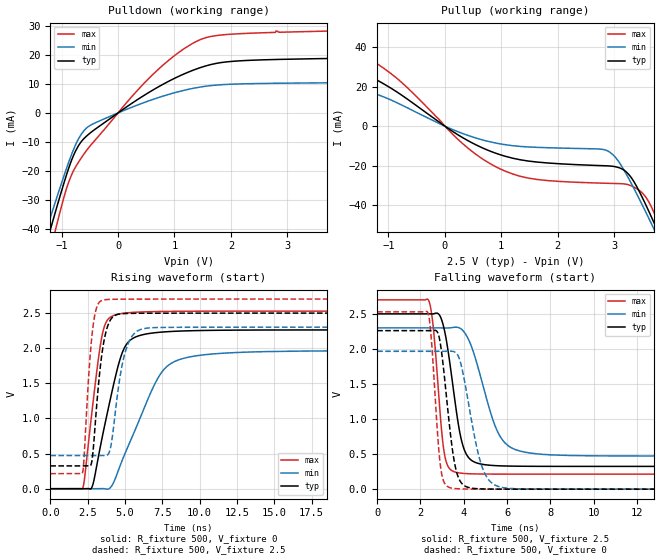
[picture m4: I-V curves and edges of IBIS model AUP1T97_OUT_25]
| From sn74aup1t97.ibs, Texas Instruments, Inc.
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[Model]   AUP1T97_OUT_25
Model_type  Output
Vref =   0
Rref =   1E6
Cref =   30p
Vmeas =   1.25
| variable   typ   min   max
C_comp   2.77pF   1.87pF   4.14pF
| C_pullup   3.12pF   1.87pF   4.14pF
| C_pulldown   2.42pF   2.13pF   2.99pF
[Temperature Range]   40   100   -40
| Ambient temperature   25   85   -40
[Voltage range]   2.5   2.3   2.7
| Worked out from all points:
|   slope of the pulldown table from 0 to 0.375 V, typ, clamps not added: 75.2 ohm
|   slope of the pullup table from 0 to 0.375 V, typ, clamps not added: 55.1 ohm
|   rising waveform, R_fixture 500, V_fixture 0: 20-80 % time 1.4ns typ, 2.41ns min, 859ps max; typ from 0 V to 2.26 V
|   falling waveform, R_fixture 500, V_fixture 2.5: 20-80 % time 621ps typ, 1.07ns min, 392ps max; typ from 2.5 V to 0.325 V
|   rising waveform, R_fixture 500, V_fixture 2.5: 20-80 % time 611ps typ, 791ps min, 469ps max; typ from 0.325 V to 2.5 V
|   falling waveform, R_fixture 500, V_fixture 0: 20-80 % time 497ps typ, 750ps min, 332ps max; typ from 2.26 V to 0 V
[Pulldown]
| AUP1T97_OUT_25
|   Voltage   I(typ)   I(min)   I(max)
-3.6V     -214mA     -193.5mA   -239.7mA
-1.26V    -44.55mA   -39.92mA   -52.42mA
-1.205V   -40.74mA   -36.52mA   -48.02mA
-1.115V   -34.57mA   -31.02mA   -40.91mA
-800mV    -15.22mA   -13.22mA   -20.4mA
-685mV    -10.84mA   -8.445mA   -16.54mA
-540mV    -7.689mA   -4.911mA   -12.5mA
675mV     8.558mA    5.038mA    14.35mA
1.105V    12.9mA     7.5mA      21.28mA
1.52V     16.03mA    9.129mA    25.76mA
2.585V    18.34mA    10.19mA    27.69mA
7.2V      19.61mA    10.73mA    29.61mA
[Pullup]
| AUP1T97_OUT_25
|   Voltage   I(typ)   I(min)   I(max)
-3.6V     37.28mA    23.5mA     50.35mA
-2.355V   24.65mA    15.21mA    35.57mA
-1.425V   26.01mA    17.2mA     35.58mA
-760mV    15.58mA    10.63mA    21.96mA
405mV     -7.279mA   -4.651mA   -11.04mA
1.05V     -15.07mA   -9.293mA   -22.54mA
2.845V    -20.04mA   -12.07mA   -28.88mA
3.17V     -22.17mA   -22.09mA   -29.2mA
3.455V    -33.67mA   -37.48mA   -32.73mA
3.685V    -47.61mA   -50.92mA   -42.5mA
3.82V     -56.28mA   -59.04mA   -51.47mA
7.2V      -294.7mA   -278.7mA   -311.5mA
[Ramp]
| AUP1T97_OUT_25
| variable   typ   min   max
dV/dt_r   1.36/1.41E-09   1.18/2.41E-09   1.52/8.61E-10
dV/dt_f   1.31/6.28E-10   1.10/1.07E-09   1.50/3.97E-10
R_load = 500
[Rising Waveform]
| AUP1T97_OUT_25
R_fixture =   500
C_fixture =   0
L_fixture =   0
V_fixture =   0
V_fixture_min = 0
V_fixture_max = 0
|   Time   V(typ)   V(min)   V(max)
0s        19.04nV    76.96nV    1.464nV
2.18ns    -12.02uV   435.7nV    11.67mV
2.81ns    31.98mV    -14uV      1.128V
3.435ns   685.6mV    1.468mV    2.14V
4.315ns   1.55V      122.9mV    2.471V
4.86ns    1.956V     425.6mV    2.497V
5.43ns    2.126V     710.7mV    2.509V
7.33ns    2.227V     1.616V     2.523V
8.865ns   2.245V     1.853V     2.526V
34.99ns   2.261V     1.966V     2.528V
[Falling Waveform]
| AUP1T97_OUT_25
R_fixture =   500
C_fixture =   0
L_fixture =   0
V_fixture =   2.5
V_fixture_min = 2.3
V_fixture_max = 2.7
|   Time   V(typ)   V(min)   V(max)
0s        2.5V       2.3V       2.7V
2.38ns    2.5V       2.3V       2.69V
2.595ns   2.5V       2.3V       2.298V
3.09ns    2.288V     2.299V     534.1mV
3.665ns   1.094V     2.309V     238.6mV
3.96ns    620.3mV    2.262V     225.5mV
4.33ns    416.9mV    2.055V     219mV
5.585ns   333.8mV    804.4mV    214.8mV
6.815ns   326.6mV    528.2mV    214.4mV
34.99ns   324.7mV    472mV      214.4mV
[Rising Waveform]
| AUP1T97_OUT_25
R_fixture =   500
C_fixture =   0
L_fixture =   0
V_fixture =   2.5
V_fixture_min = 2.3
V_fixture_max = 2.7
|   Time   V(typ)   V(min)   V(max)
0s        324.7mV    472mV      214.4mV
2.155ns   324.7mV    472mV      224.1mV
2.82ns    440.6mV    472mV      2.235V
3.09ns    1.137V     472mV      2.569V
3.47ns    1.935V     472.9mV    2.682V
4.04ns    2.406V     586.3mV    2.696V
4.655ns   2.487V     1.569V     2.698V
5.08ns    2.494V     1.986V     2.699V
6.155ns   2.498V     2.274V     2.699V
34.99ns   2.5V       2.3V       2.7V
[Falling Waveform]
| AUP1T97_OUT_25
R_fixture =   500
C_fixture =   0
L_fixture =   0
V_fixture =   0
V_fixture_min = 0
V_fixture_max = 0
|   Time   V(typ)   V(min)   V(max)
0s        2.261V     1.966V     2.528V
2.345ns   2.261V     1.966V     2.515V
2.5ns     2.26V      1.966V     2.143V
2.805ns   2.225V     1.966V     725.9mV
2.93ns    2.05V      1.966V     314mV
3.42ns    694.4mV    1.967V     16.58mV
3.845ns   108.4mV    1.81V      3.901mV
4.87ns    3.385mV    296.3mV    201.8uV
5.77ns    436.8uV    24mV       27.55uV
34.99ns   16.41nV    213.8nV    -14.24nV
